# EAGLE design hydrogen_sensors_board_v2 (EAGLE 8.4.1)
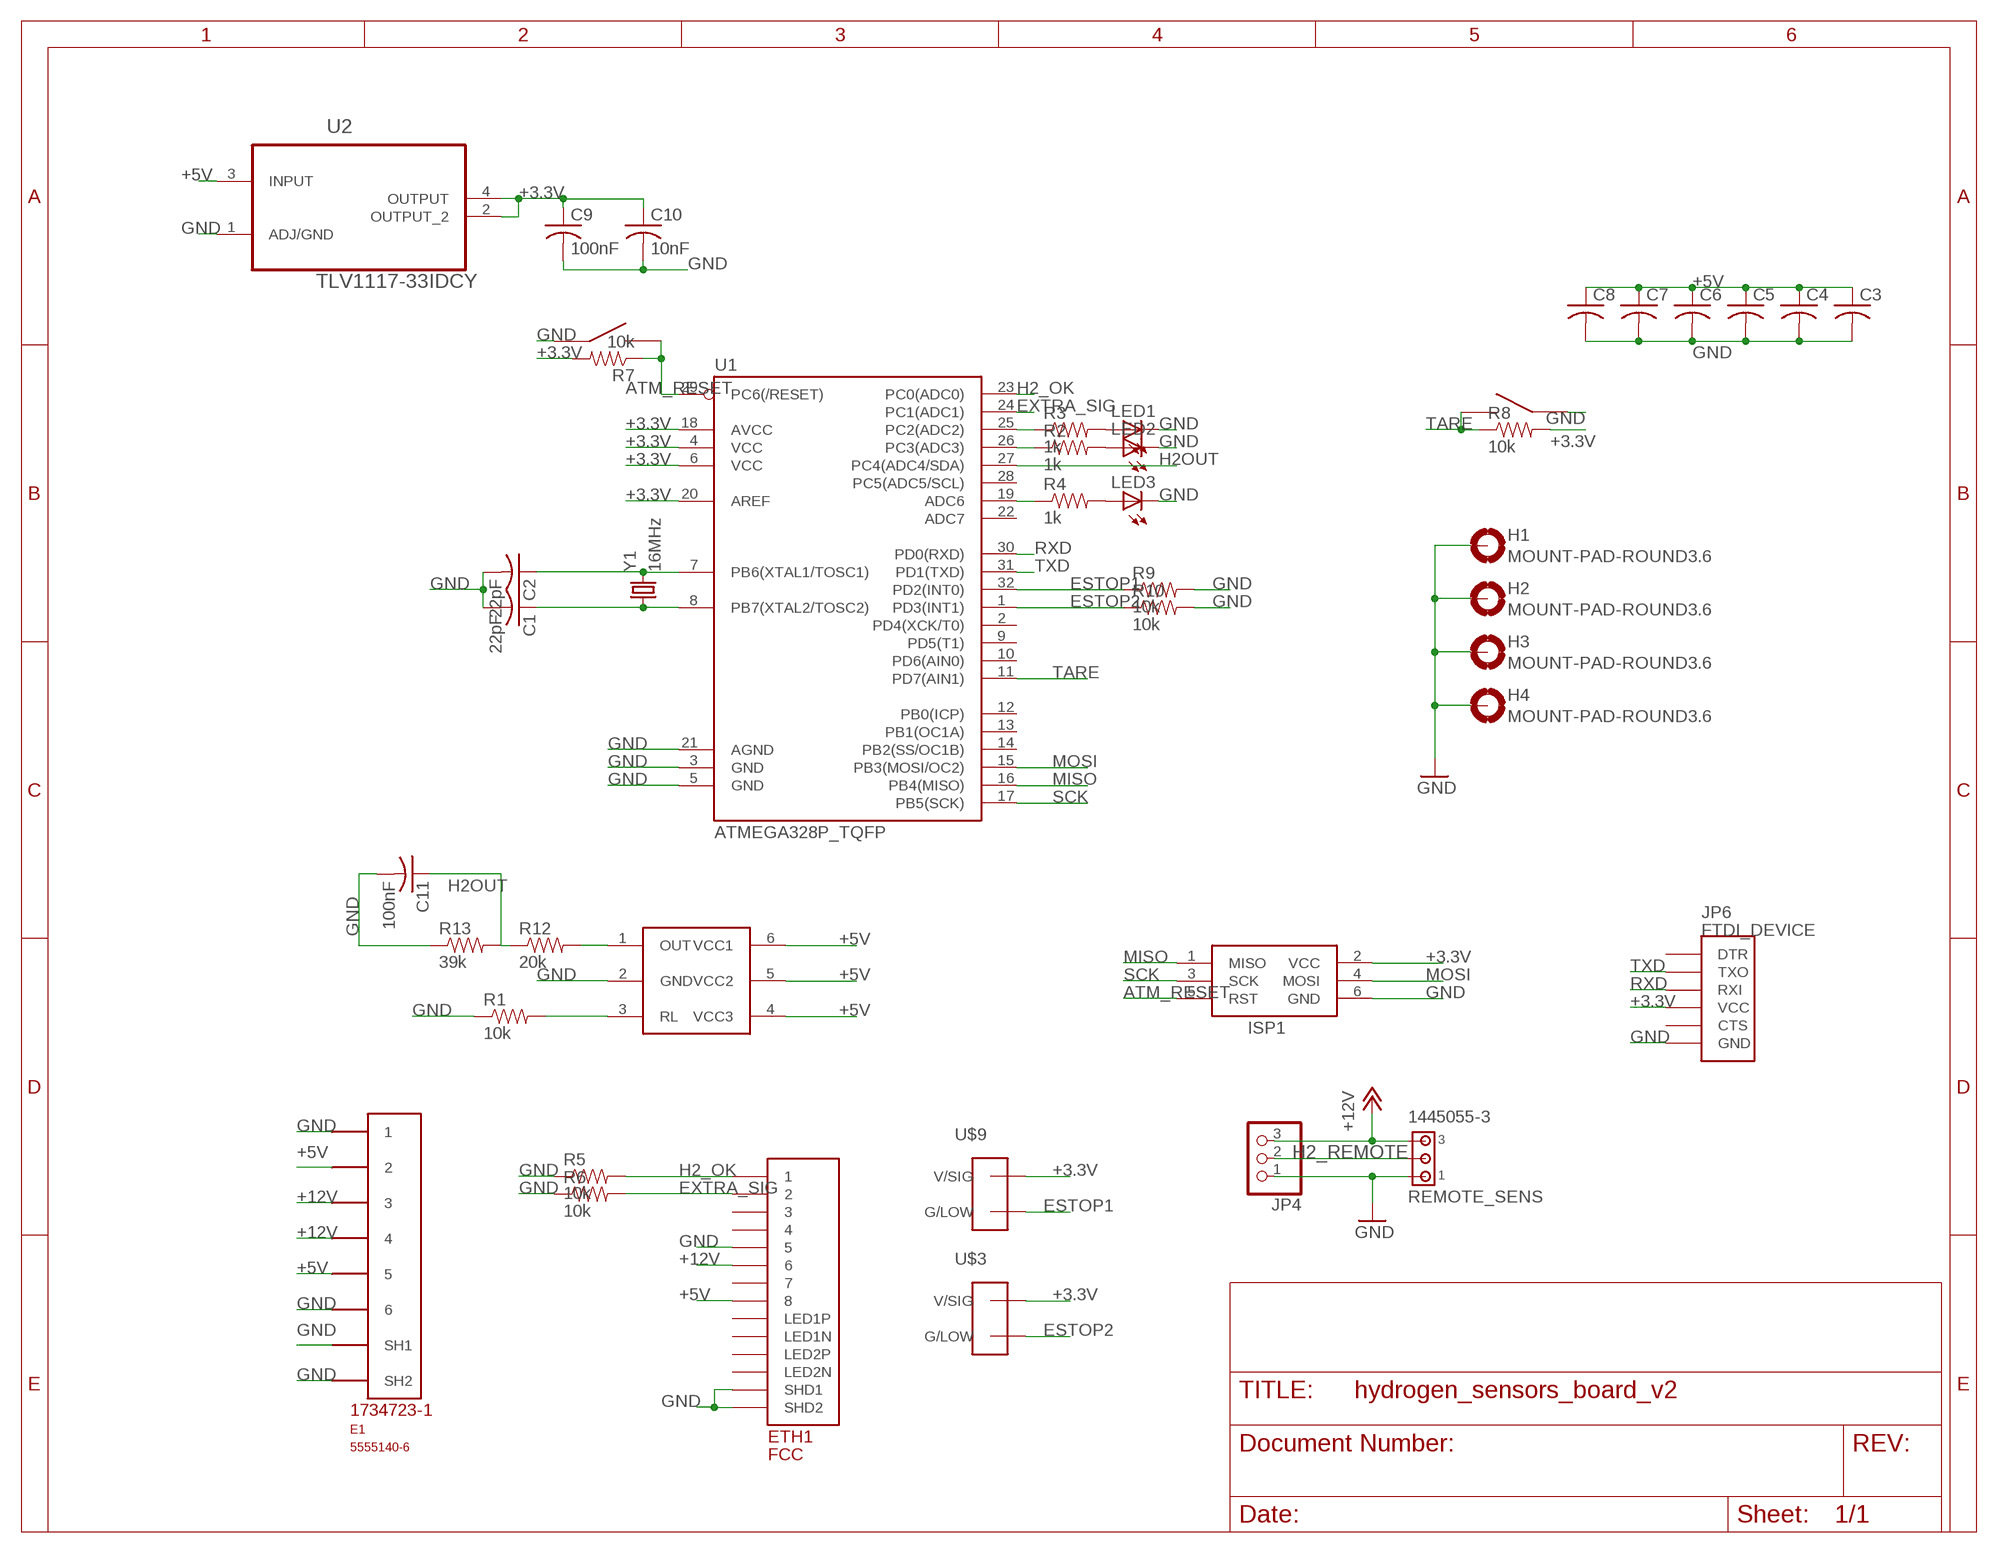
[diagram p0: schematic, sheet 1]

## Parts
C1  22pF  C-USC0603K  [C0603K]
C2  22pF  C-USC0603K  [C0603K]
C3  C-USC0603  [C0603]
C4  C-USC0603  [C0603]
C5  C-USC0603  [C0603]
C6  C-USC0603  [C0603]
C7  C-USC0603  [C0603]
C8  C-USC0603  [C0603]
C9  100nF  C-USC0603  [C0603]
C10  10nF  C-USC0603  [C0603]
C11  100nF  C-USC0603  [C0603]
E1  5555140-6  [1734723-1_RJ11]
ETH1  FCC  ETHERNET  [A122645-ND]
H1  MOUNT-PAD-ROUND3.6  [3,6-PAD]
H2  MOUNT-PAD-ROUND3.6  [3,6-PAD]
H3  MOUNT-PAD-ROUND3.6  [3,6-PAD]
H4  MOUNT-PAD-ROUND3.6  [3,6-PAD]
ISP1  AVRISP-BOX  [AVRISP-BOX]
JP4  PINHD-1X3  [1X03]
JP6  FTDI_DEVICE  [FTDI_DEVICE_SIDE]
LED1  LEDCHIPLED_0805  [CHIPLED_0805]
LED2  LEDCHIPLED_0805  [CHIPLED_0805]
LED3  LEDCHIPLED_0805  [CHIPLED_0805]
R1  10k  RESISTOR0603-RES  [0603-RES]
R2  1k  RESISTOR0603-RES  [0603-RES]
R3  1k  RESISTOR0603-RES  [0603-RES]
R4  1k  RESISTOR0603-RES  [0603-RES]
R5  10k  RESISTOR0603-RES  [0603-RES]
R6  10k  RESISTOR0603-RES  [0603-RES]
R7  10k  RESISTOR0603-RES  [0603-RES]
R8  10k  RESISTOR0603-RES  [0603-RES]
R9  10k  RESISTOR0603-RES  [0603-RES]
R10  10k  RESISTOR0603-RES  [0603-RES]
R12  20k  RESISTOR0603-RES  [0603-RES]
R13  39k  RESISTOR0603-RES  [0603-RES]
REMOTE_SENS  1445055-3  [1445055-3]
U1  ATMEGA328P_TQFP  [TQFP32-08]
U2  TLV1117-33IDCY  [SOT230P700X180-4N]
U$1  MQ-8MQ-8  [MQ-8]
U$2  EG4621CT-ND  [EG4621CT-ND]
U$3  TE770966  [2X1-MATE-N-LOCK]
U$9  TE770966  [2X1-MATE-N-LOCK]
U$10  EG4621CT-ND  [EG4621CT-ND]
Y1  16MHz  CRYSTALHC49US  [HC49US]

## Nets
+3.3V: C9.1 C10.1 ISP1.2(VCC) JP6.P$4(VCC) R7.2 R8.2 U1.4(VCC) U1.6(VCC) U1.18(AVCC) U1.20(AREF) U2.2(OUTPUT_2) U2.4(OUTPUT) U$3.CIRCUIT1(V/SIG) U$9.CIRCUIT1(V/SIG)
+5V: C3.1 C4.1 C5.1 C6.1 C7.1 C8.1 E1.2 E1.5 ETH1.P$8 U2.3(INPUT) U$1.4(VCC3) U$1.5(VCC2) U$1.6(VCC1)
+12V: E1.3 E1.4 ETH1.P$6 JP4.3 REMOTE_SENS.3
ATM_RESET: ISP1.5(RST) R7.1 U1.29(PC6(/RESET)) U$10.P$3 U$10.P$4
ESTOP1: R9.1 U1.32(PD2(INT0)) U$9.CIRCUIT2(G/LOW)
ESTOP2: R10.1 U1.1(PD3(INT1)) U$3.CIRCUIT2(G/LOW)
EXTRA_SIG: ETH1.P$2 R6.2 U1.24(PC1(ADC1))
GND: C1.2 C2.2 C3.2 C4.2 C5.2 C6.2 C7.2 C8.2 C9.2 C10.2 C11.2 E1.1 E1.6 E1.SH1 E1.SH2 ETH1.P$5 ETH1.P$13(SHD1) ETH1.P$14(SHD2) H1.B3,6(MOUNT) H2.B3,6(MOUNT) H3.B3,6(MOUNT) H4.B3,6(MOUNT) ISP1.6(GND) JP4.1 JP6.P$6(GND) LED1.C LED2.C LED3.C R1.1 R5.1 R6.1 R9.2 R10.2 R13.1 REMOTE_SENS.1 U1.3(GND) U1.5(GND) U1.21(AGND) U2.1(ADJ/GND) U$1.2(GND) U$2.P$1 U$2.P$2 U$10.P$1 U$10.P$2
H2_OK: ETH1.P$1 R5.2 U1.23(PC0(ADC0))
H2_REMOTE: JP4.2 REMOTE_SENS.2
H2OUT: C11.1 R12.1 R13.2 U1.27(PC4(ADC4/SDA))
MISO: ISP1.1(MISO) U1.16(PB4(MISO))
MOSI: ISP1.4(MOSI) U1.15(PB3(MOSI/OC2))
N$1: C2.1 U1.7(PB6(XTAL1/TOSC1)) Y1.2
N$2: R1.2 U$1.3(RL)
N$3: C1.1 U1.8(PB7(XTAL2/TOSC2)) Y1.1
N$4: R3.1 U1.25(PC2(ADC2))
N$5: R2.1 U1.26(PC3(ADC3))
N$6: R4.1 U1.19(ADC6)
N$7: LED1.A R3.2
N$8: LED2.A R2.2
N$9: LED3.A R4.2
N$10: R12.2 U$1.1(OUT)
RXD: JP6.P$3(RXI) U1.30(PD0(RXD))
SCK: ISP1.3(SCK) U1.17(PB5(SCK))
TARE: R8.1 U1.11(PD7(AIN1)) U$2.P$3 U$2.P$4
TXD: JP6.P$2(TXO) U1.31(PD1(TXD))
Unconnected: ETH1.P$3 ETH1.P$4 ETH1.P$7 ETH1.P$9(LED1N) ETH1.P$10(LED1P) ETH1.P$11(LED2N) ETH1.P$12(LED2P) JP6.P$1(DTR) JP6.P$5(CTS) U1.2(PD4(XCK/T0)) U1.9(PD5(T1)) U1.10(PD6(AIN0)) U1.12(PB0(ICP)) U1.13(PB1(OC1A)) U1.14(PB2(SS/OC1B)) U1.22(ADC7) U1.28(PC5(ADC5/SCL))

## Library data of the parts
C1-C11 = adafruit:C-US: CAPACITOR, American symbol
E1 = 5555140-6 RJ11:5555140-6
ETH1 = ETHERNET:ETHERNET: Ethernet port with 2 leds. digikey number A122645-ND
H1-H4 = holes:MOUNT-PAD-ROUND: MOUNTING PAD, round
ISP1 = adafruit:AVRISP: AVR ISP HEADER Standard 6 pin header for AVR programming
JP4 = pinhead:PINHD-1X3: PIN HEADER
JP6 = SparkFun-Connectors:FTDI_DEVICE: Connector which mates to FTDI basic or FTDI cable.
LED1-LED3 = adafruit:LED: LED
R1 R5 R6 R9 R10 R12 R13 = SparkFun-Passives:RESISTOR: Resistor
R2-R4 R7 R8 = SparkFun-Resistors:RESISTOR: Resistor
REMOTE_SENS = con-amp:1445055-3: Micro MATE-N-LOK Connectors grid 1.5 mm Source: ENG_CD_1445055_A.pdf
U1 = SparkFun-DigitalIC:ATMEGA328P_TQFP; PROD_ID: IC-09069
U2 = Texas Instruments_By_element14_Batch_1:TLV1117-33IDCY: V REG, LDO, 3.3V, 0.8A; MPN: TLV1117-33IDCY; OC_FARNELL: 1703385; OC_NEWARK: 67K8522; PACKAGE: SOT-223-3; SUPPLIER: TEXAS INSTRUMENTS
U$1 = donny_library:MQ-8
U$2 U$10 = EG4621CT-ND:EG4621CT-ND: surface mount push putton digikey number EG4621CT-ND
U$3 U$9 = Shell2013:TE770966
Y1 = SparkFun-FreqCtrl:CRYSTAL: Various standard crystals. Proven footprints.

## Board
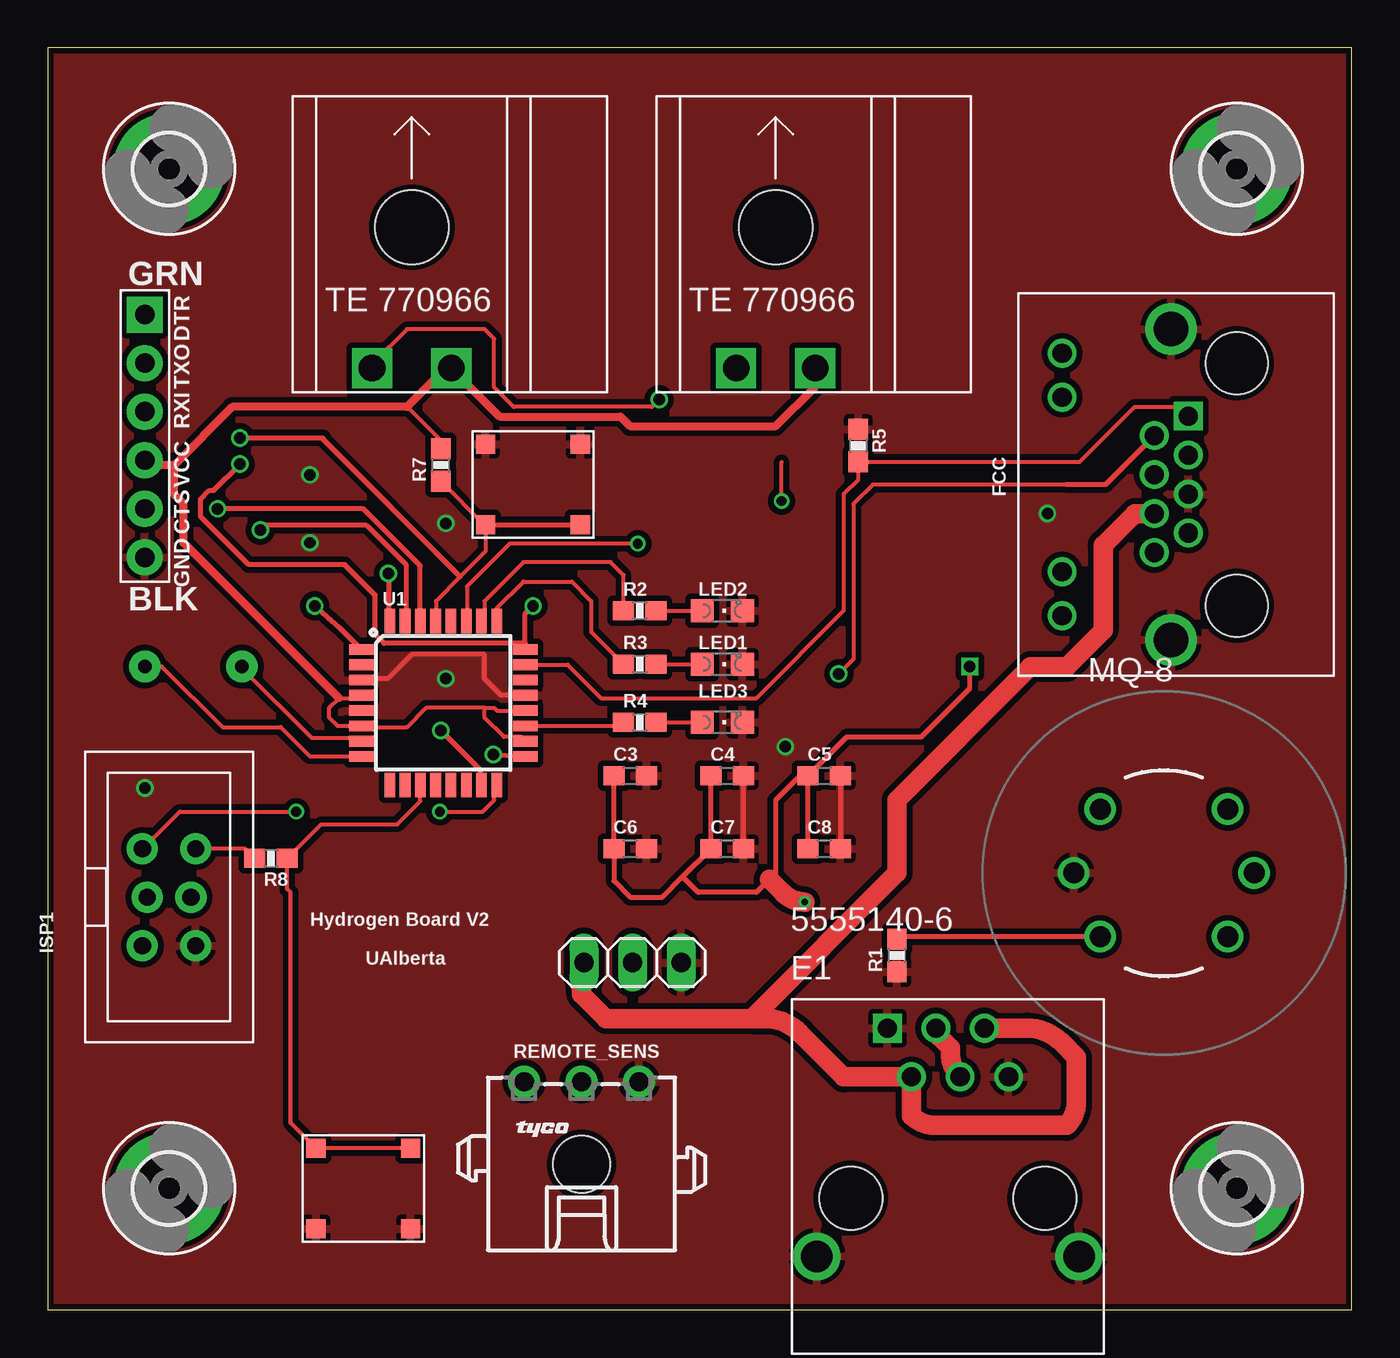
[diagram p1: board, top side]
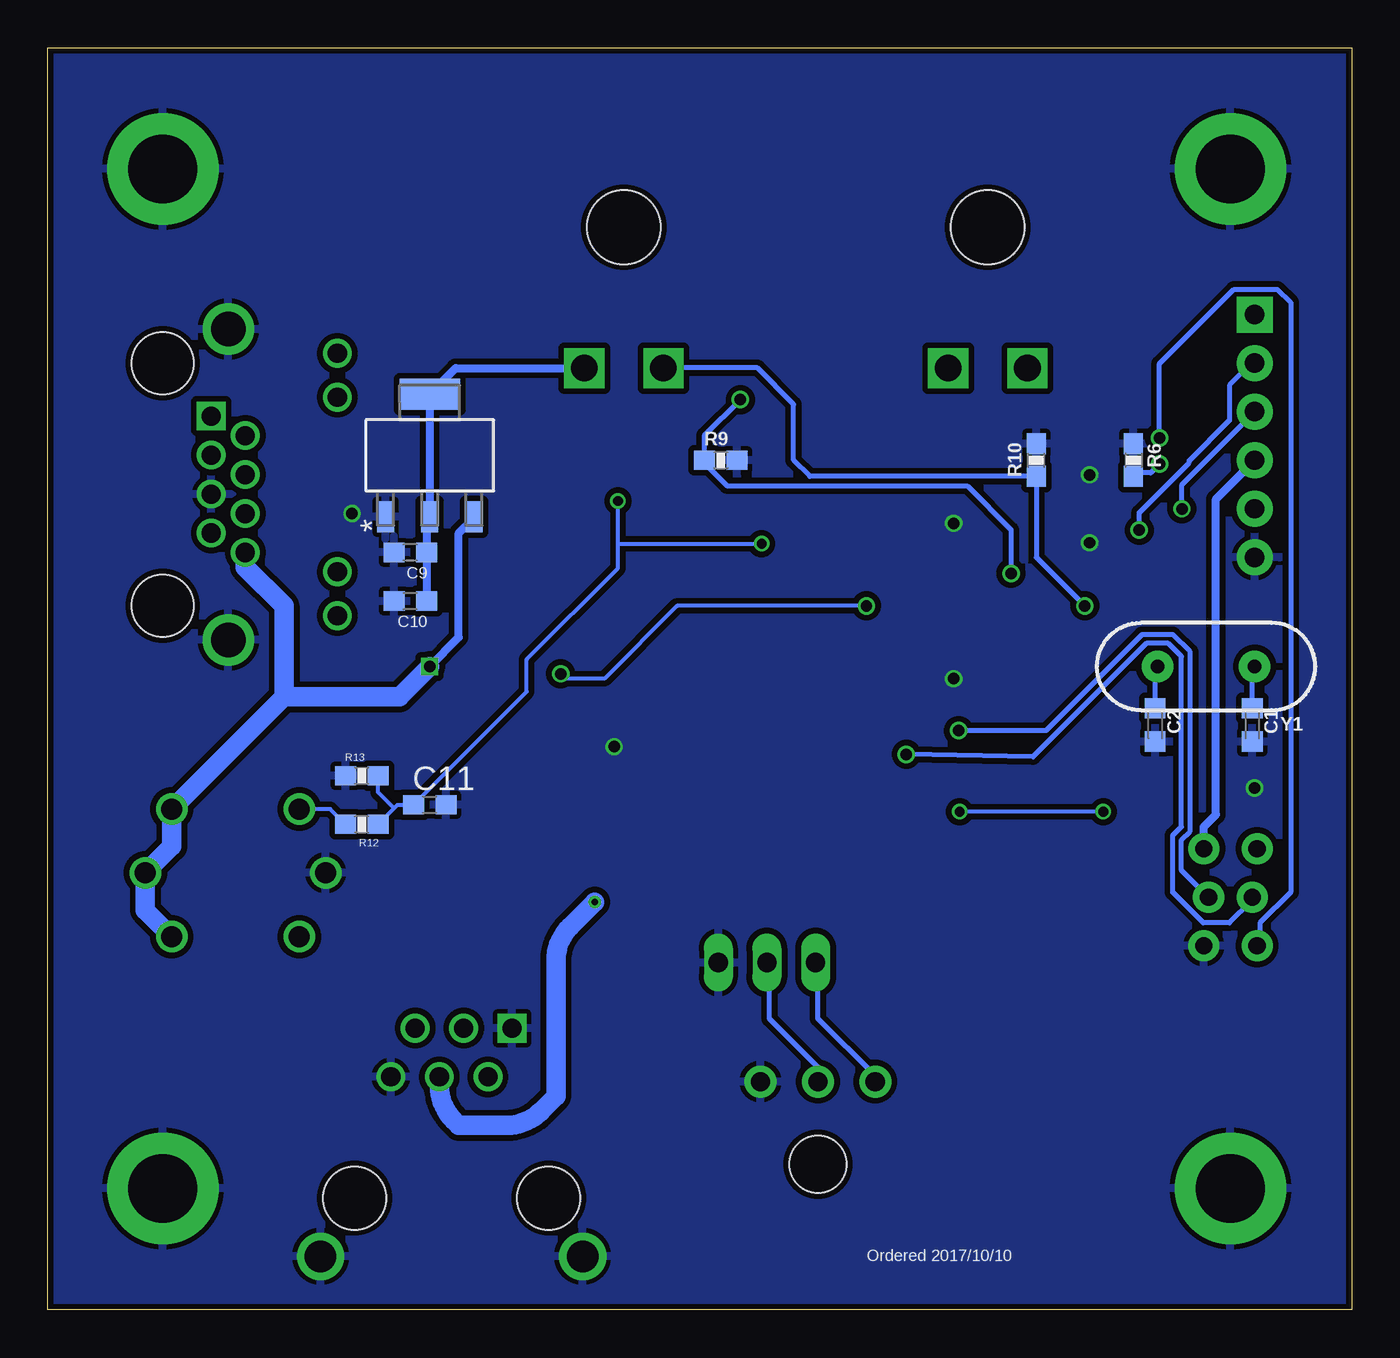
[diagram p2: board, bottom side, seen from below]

Size 68.25 x 66.03 mm. Coordinates in mm from the lower left corner, seen from the top.
Outline: 0,0 68.25,0 68.25,66.03 0,66.03 0,0
Copper layers (1*16): Top 0.035mm / dielectric 1.5mm / Bottom 0.035mm
Design rules "SeeedStudio_2layer_DRU_no_angle_20140221": minimum track width 6mil, minimum drill 12mil, track to track 6mil, track to pad 6mil, pad to pad 6mil, via to via 6mil, smd to smd 0mil, copper to edge 10mil, drill to drill 10mil, minimum pad ring 10mil, minimum via ring 6mil, stop-mask expansion 2mil, vias tented up to drill 100mil, thermal gap 10mil

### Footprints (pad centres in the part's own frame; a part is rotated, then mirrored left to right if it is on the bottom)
C0603K = smd 1.05 x 1.08: 1 -0.875,0; 2 0.875,0
C0603 = smd 1.1 x 1: 1 -0.85,0; 2 0.85,0
1734723-1_RJ11 = drill 1 square: 1 -3.81,2.54 | drill 1: 2 -1.27,2.54; 3 1.27,2.54; 4 -2.54,0; 5 0,0; 6 2.54,0 | drill 1.65: SH1 -7.5,-9.4; SH2 6.22,-9.4 | hole 3.3: -5.72,-6.35; 4.44,-6.35
A122645-ND = drill 1 square: P$1 3.58,2.54 | drill 1: P$2 2.56,4.32; P$3 1.54,2.54; P$4 0.52,4.32; P$5 -0.5,2.54; P$6 -1.52,4.32; P$7 -2.54,2.54; P$8 -3.56,4.32; P$9 -6.86,9.14; P$10 -4.57,9.14; P$11 4.57,9.14; P$12 6.86,9.14 | drill 1.8: P$13 -8.13,3.43; P$14 8.13,3.43 | hole 3.25: -6.35,0; 6.35,0
3,6-PAD = drill 3.6 pad 5.842: B3,6 0,0
AVRISP-BOX = drill 0.9 pad 1.626: 1 -1.397,2.54; 2 1.397,2.54; 3 -1.143,0; 4 1.143,0; 5 -1.397,-2.54; 6 1.397,-2.54
1X03 = drill 1.016 long: 1 -2.54,0; 2 0,0; 3 2.54,0
FTDI_DEVICE_SIDE = drill 1.016 pad 1.88 square: P$1 -6.35,0 | drill 1.016 pad 1.88: P$2 -3.81,0; P$3 -1.27,0; P$4 1.27,0; P$5 3.81,0; P$6 6.35,0
CHIPLED_0805 = smd 1.2 x 1.2: A 0,-1.05; C 0,1.05
0603-RES = smd 1.1 x 1: 1 -0.85,0; 2 0.85,0
1445055-3 = drill 1 pad 1.676: 1 3,4.32; 2 0,4.32; 3 -3,4.32 | hole 3: 0,0
TQFP32-08 = smd 1.27 x 0.559: 1 -4.293,2.8; 2 -4.293,2; 3 -4.293,1.2; 4 -4.293,0.4; 5 -4.293,-0.4; 6 -4.293,-1.2; 7 -4.293,-2; 8 -4.293,-2.8; 17 4.293,-2.8; 18 4.293,-2; 19 4.293,-1.2; 20 4.293,-0.4; 21 4.293,0.4; 22 4.293,1.2; 23 4.293,2; 24 4.293,2.8 | smd 0.559 x 1.27: 9 -2.8,-4.293; 10 -2,-4.293; 11 -1.2,-4.293; 12 -0.4,-4.293; 13 0.4,-4.293; 14 1.2,-4.293; 15 2,-4.293; 16 2.8,-4.293; 25 2.8,4.293; 26 2,4.293; 27 1.2,4.293; 28 0.4,4.293; 29 -0.4,4.293; 30 -1.2,4.293; 31 -2,4.293; 32 -2.8,4.293
SOT230P700X180-4N = smd 1.626 x 0.889: 1 -3.2,2.311; 2 -3.2,0; 3 -3.2,-2.311 | smd 1.626 x 3.175: 4 3.2,0
MQ-8 = drill 1.1: 1 -3.337,3.337; 2 -4.72,0; 3 -3.337,-3.337; 4 3.337,-3.337; 5 4.72,0; 6 3.337,3.337
EG4621CT-ND = smd 1 x 1: P$1 -2.475,2.1; P$2 2.475,2.1; P$3 -2.475,-2.1; P$4 2.475,-2.1
2X1-MATE-N-LOCK = drill 1.4 square: CIRCUIT1 -2.07,14.23; CIRCUIT2 2.07,14.23 | hole 3.86: 0,6.86
HC49US = drill 0.7 pad 1.651: 1 -2.54,0; 2 2.54,0

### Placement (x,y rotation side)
C1  5.21,30.61 270 bottom
C2  10.29,30.61 270 bottom
C3  30.48,27.94 0 top
C4  35.56,27.94 0 top
C5  40.64,27.94 0 top
C6  30.48,24.13 0 top
C7  35.56,24.13 0 top
C8  40.64,24.13 0 top
C9  49.28,39.62 180 bottom
C10  49.28,37.08 180 bottom
C11  48.26,26.42 0 bottom
E1  47.75,12.19 0 top
ETH1  62.23,43.18 90 top
H1  6.35,59.69 0 top
H2  62.23,59.69 0 top
H3  62.23,6.35 0 top
H4  6.35,6.35 0 top
ISP1  6.35,21.59 0 top
JP4  30.61,18.16 180 top
JP6  5.08,45.72 270 top
LED1  35.31,33.78 270 top
LED2  35.31,36.58 270 top
LED3  35.31,30.73 270 top
R1  44.45,18.54 90 top
R2  30.99,36.58 0 top
R3  30.99,33.78 0 top
R4  30.99,30.73 0 top
R5  42.42,45.21 270 top
R6  11.43,44.45 270 bottom
R7  20.57,44.2 90 top
R8  11.68,23.62 180 top
R9  33.02,44.45 0 bottom
R10  16.51,44.45 90 bottom
R12  51.82,25.4 180 bottom
R13  51.82,27.94 0 bottom
REMOTE_SENS  27.94,7.62 0 top
U1  20.7,31.75 0 top
U2  48.26,44.7 90 bottom
U$1  58.42,22.86 0 top
U$2  16.51,6.35 180 top
U$3  38.1,63.5 180 top
U$9  19.05,63.5 180 top
U$10  25.4,43.18 0 top
Y1  7.62,33.66 180 bottom

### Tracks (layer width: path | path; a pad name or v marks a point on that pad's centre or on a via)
+3.3V
  Top 0.203: U1.4 16.26,32 15.24,32 14.73,31.5 14.73,30.99 15.17,30.55 U1.6 16.48,30.48 18.8,30.48 19.81,31.5 22.86,31.5 | 22.86,31.5 23.37,31.5 23.51,31.35 U1.20 | U1.18 24.77,29.97 23.88,29.97 22.86,30.99 22.86,31.5 | 18.8,47.24 20.57,45.47 R7.2 | R8.2 10.33,24.13 ISP1.2
  Top 0.406: 6.6,44.2 9.65,47.24 18.8,47.24 20.82,49.27 U$9.CIRCUIT1 23.65,46.74 29.97,46.74 30.48,46.23 38.1,46.23 40.17,48.3 U$3.CIRCUIT1 | 6.6,44.2 5.33,44.2 JP6.P$4 | 15.24,32 7.11,40.13 7.11,42.16 6.6,42.67 6.6,44.2
  Bottom 0.406: ISP1.2 7.75,25.27 7.11,25.91 7.11,42.42 JP6.P$4 | U$3.CIRCUIT1 46.89,49.27 U2.4 U2.2 48.43,41.34 C9.1 C10.1
+5V  (via drill 0.35, 0.6)
  Top 0.254: C5.1 41.82,29.97 45.72,29.97 48.26,32.51 v48.26,33.66 | C8.1 C5.1 | C4.1 C7.1 33.23,22.65 | C3.1 C6.1 29.63,22.44 30.48,21.59 32.17,21.59 33.23,22.65 | C5.1 39.37,27.94 38.1,26.67 38.1,22.86 37.77,22.53 37.08,21.84 34.04,21.84 33.23,22.65
  Top 1.016: v39.62,21.34 arc-45 38.49,21.81 37.77,22.53 | E1.2 arc45 46.66,14.3 47.24,13.72 47.24,13.42 arc45 E1.5
  Bottom 0.406: v48.26,33.66 46.74,35.18 46.74,40.64 45.95,41.43 U2.3
  Bottom 1.016: ETH1.P$8 57.91,38.86 55.88,36.83 55.88,32.08 | 55.88,32.08 U$1.6 61.76,24.24 U$1.5 63.14,20.91 U$1.4 | 55.88,32.08 49.84,32.08 v48.26,33.66 | E1.5 47.75,11.72 arc-45 47.01,9.92 46.74,9.65 44.23,9.65 arc-45 42.44,10.4 41.66,11.18 41.66,18.25 arc45 40.91,20.05 v39.62,21.34
+12V
  Top 1.016: ETH1.P$6 56.9,41.66 55.24,40.01 55.24,35.56 53.34,33.66 51.44,33.66 44.45,26.67 44.45,22.86 36.83,15.24 | 36.83,15.24 29.21,15.24 27.94,16.51 27.94,18.03 JP4.3 | 36.83,15.24 37.56,15.24 arc-45 39.35,14.5 41.66,12.19 E1.4 45.21,10.16 arc45 46.44,9.65 53.34,9.65 arc45 53.85,10.88 53.85,13.21 53.07,13.99 arc45 51.27,14.73 E1.3
  Bottom 0.254: REMOTE_SENS.3 24.94,12.24 27.94,15.24 27.94,18.03 JP4.3
ATM_RESET  (via drill 0.61)
  Top 0.203: U1.29 20.32,36.06 20.32,37.08 21.59,38.35 22.93,39.69 U$10.P$3 22.84,41.08 R7.1
  Top 0.254: U$10.P$3 U$10.P$4 | v10.06,45.62 14.4,45.62 14.4,45.54 21.59,38.35
  Bottom 0.254: v10.06,45.62 10.06,49.51 6.17,53.39 3.89,53.39 3.2,52.7 3.2,21.84 4.8,20.24 4.8,19.1 ISP1.5
ESTOP1  (via drill 0.6, 0.61)
  Top 0.203: v32,47.62 31.62,47.24 24.38,47.24 23.37,48.26 23.37,50.8 22.86,51.31 18.8,51.31 16.98,49.49 U$9.CIRCUIT2
  Top 0.254: v17.83,38.53 17.83,36.25 U1.32
  Bottom 0.254: v32,47.62 33.87,45.76 R9.1 33.83,44.25 32.69,43.1 20.12,43.1 17.83,40.82 v17.83,38.53
ESTOP2  (via drill 0.6)
  Top 0.254: v13.97,36.83 15.24,35.72 U1.1
  Bottom 0.254: U$3.CIRCUIT2 31.11,49.28 29.21,47.37 29.21,44.45 28.36,43.6 R10.1 16.51,39.37 v13.97,36.83
EXTRA_SIG  (via drill 0.6, 0.61)
  Top 0.203: 53.34,43.18 43.18,43.18 42.16,42.16 42.16,34.04 v41.4,33.27
  Top 0.254: U1.24 24.99,34.87 | 24.99,34.87 24.99,36.42 v25.4,36.83 | 53.34,43.18 55.35,43.18 ETH1.P$2 | v10.06,44.25 8.69,42.88 8.46,42.88 8,42.42 8,41.5 10.52,38.99 15.54,38.99 17.14,37.39 17.14,35.33 17.6,34.87 24.99,34.87
  Bottom 0.203: v25.4,36.83 35.31,36.83 39.12,33.02 41.15,33.02 v41.4,33.27
  Bottom 0.254: v10.06,44.25 10.52,43.79 11.43,43.79 R6.2
GND  (via drill 0.6 pad 0.75)
  Top 0.254: U1.21 23.73,32.15 22.86,33.02 22.86,34.29 19.05,34.29 17.78,33.02 16.48,33.02 U1.3 | C5.2 C8.2 | C7.2 C4.2
  other vias: 5.08,27.3 52.32,41.66 38.61,29.46 13.72,43.69 13.72,40.13 20.83,41.15 20.83,33.02
  pour Top (isolate 0.305): 0,0 0,66.04 68.58,66.04 68.58,0
  pour Bottom (isolate 0.305): 0,0 0,66.04 70.48,66.04 70.48,0
H2_OK
  Top 0.203: U1.23 27.21,33.75 28.96,32 37.08,32 41.66,36.58 41.66,42.67 42.42,43.43 R5.2 54.01,44.36 56.9,47.24 59.21,47.24 ETH1.P$1
H2_REMOTE
  Bottom 0.254: REMOTE_SENS.2 27.94,12.7 30.48,15.24 30.48,18.03 JP4.2
H2OUT  (via drill 0.51)
  Top 0.203: v38.41,42.32 38.41,44.35 | v30.89,40.08 24.18,40.08 21.95,37.85 21.95,36.22 U1.27
  Bottom 0.203: 38.41,40.08 v38.41,42.32 | 38.41,40.08 v30.89,40.08 | R12.1 50.12,26.25 | 50.12,26.25 49.95,26.42 C11.1 43.18,32.35 43.18,34.04 38.41,38.81 38.41,40.08 | 50.12,26.25 50.97,27.09 R13.2
MISO  (via drill 0.51)
  Top 0.203: v20.52,26.06 22.76,26.06 23.37,26.67 23.37,27.28 U1.16 | v13.01,26.06 6.91,26.06 5.08,24.23 ISP1.1
  Bottom 0.203: v13.01,26.06 v20.52,26.06
MOSI  (via drill 0.61)
  Top 0.254: v20.57,30.3 22.63,28.25 22.63,27.56 U1.15
  Bottom 0.254: v20.57,30.3 16,30.3 10.97,35.33 9.37,35.33 8.46,34.42 8.46,25.04 8.91,24.59 8.91,22.99 7.54,21.61 ISP1.4
N$1
  Top 0.203: U1.7 16.26,29.92 13.82,29.92 10.16,33.58 Y1.2
  Bottom 0.254: C2.1 10.29,33.53 Y1.2
N$2
  Top 0.254: U$1.3 44.58,19.52 R1.2
  Bottom 0.203: 55.07,19.56 U$1.3
N$3
  Top 0.203: Y1.1 5.97,33.66 9.14,30.48 12.19,30.48 13.72,28.96 U1.8
  Bottom 0.254: C1.1 5.21,33.53 Y1.1
N$4
  Top 0.203: U1.25 23.5,36.71 24.89,38.1 27.43,38.1 28.45,37.08 28.45,35.47 R3.1
N$5
  Top 0.203: R2.1 30.14,38.44 29.46,39.12 24.89,39.12 22.86,37.08 22.86,36.2 U1.26
N$6
  Top 0.203: U1.19 29.95,30.55 R4.1
N$7
  Top 0.203: R3.2 LED1.A
N$8
  Top 0.203: R2.2 LED2.A
N$9
  Top 0.203: R4.2 LED3.A
N$10
  Bottom 0.203: R12.2 53.46,26.2 U$1.1
RXD  (via drill 0.6)
  Top 0.254: U1.30 19.5,38.92 16.51,41.91 v8.89,41.91
  Bottom 0.254: v8.89,41.91 8.89,43.18 JP6.P$3
SCK  (via drill 0.61)
  Top 0.254: v23.32,29.06 24.92,28.93 U1.17
  Bottom 0.254: v23.32,29.06 16.69,28.93 10.74,34.87 9.6,34.87 8.91,34.19 8.91,25.27 9.37,24.82 9.37,21.84 7.77,20.24 6.4,20.24 5.26,21.39 ISP1.3
TARE
  Top 0.203: U$2.P$3 U$2.P$4 12.7,9.79 12.7,21.84 12.53,22.01 R8.1 14.31,25.4 18.29,25.4 19.5,26.61 U1.11
TXD  (via drill 0.61)
  Top 0.254: U1.31 18.75,36.25 18.75,38.99 16.69,41.05 11.38,41.05 v11.12,40.79
  Bottom 0.254: JP6.P$2 5.26,49.51 6.4,48.36 6.4,46.53 8.51,44.42 8.51,44.32 11.12,41.71 v11.12,40.79

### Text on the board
tPlace: Hydrogen Board V2 | UAlberta
bPlace: Ordered 2017/10/10

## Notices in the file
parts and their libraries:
SparkFun-DigitalIC: Licensing: Creative Commons ShareAlike 4.0 International - https://creativecommons.org/licenses/by-sa/4.0
SparkFun: Licensing: CC v3.0 Share-Alike You are welcome to use this library for commercial purposes.
